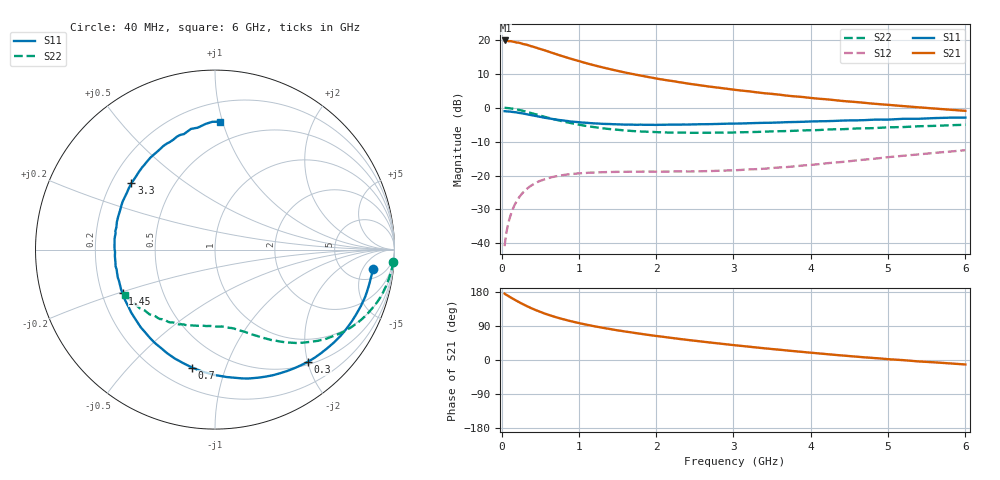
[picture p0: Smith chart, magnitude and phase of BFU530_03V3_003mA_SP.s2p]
! Filename:  P:\Prog\Test\Noise\ATS_data\Testdata_Net\03 Spar\BFU530_APG2013_40_A05_03p3V_003mA_SP_CM01_D.s2p
! Date/Time: Fri 26/Apr/2013 13:03:17
! BFU530_APG2013_40_A05_03p3V_1to25mA_SP_CM01_Bias3_R.s2p
! MDIF S-parameter v. bias file
! BFU530_APG2013_40_A05_03p3V_1to25mA_SP_CM01
! Date/time Wed Apr 24 18:17:07 2013
! VAR V_out= 3.3000
! VAR I_out= 2.9950
! VAR V_in= 0.8102
! VAR I_in= 0.0328
! Device data file deembeded for feedlines and parallel
! Original file: \03 Spar\BFU530_APG2013_40_A05_03p3V_003mA_SP_CM01_R.s2p
! Feed-files: PR047V01_250413_Feed1.s2p, PR047V01_250413_Feed2.s2p
! Parallel-file: PR047V01_250413_Par.s2p
# MHz S MA R 50
!  Freq-MHz  S11-mag  S11-arg  S21-mag  S21-arg  S12-mag  S12-arg  S22-mag  S22-arg
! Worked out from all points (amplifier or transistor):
!   98 points, 40 MHz to 6 GHz, reference 50 ohm
!   highest |S21| = 19.8 dB at 50 MHz (marker M1)
!   |S21| within 3 dB of that: start of sweep to 570 MHz
!   unconditionally stable (mu >= 1): 2.566 GHz to 4.777 GHz
!   at 300 MHz: K = 0.14, MSG = 21.6 dB, |S12| = -24.5 dB
!   at 1.6 GHz: K = 0.67, MSG = 14.6 dB, |S12| = -18.9 dB
!   at 6 GHz: K = 0.85, MSG = 5.8 dB, |S12| = -12.5 dB
!   S11 on the Smith chart (normalised r, x): 40 MHz: 8, -8; 300 MHz: 0.55, -2.00; 700 MHz: 0.32, -0.77; 1.45 GHz: 0.29, -0.21; 3.3 GHz: 0.28, +0.32; 6 GHz: 0.34, +0.98
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40  0.8866 -7.1  9.759 175.1  0.009105 85.7  0.9938 -3.9
50  0.8846 -8.9  9.775 173.1  0.01136 84.5  0.9941 -5.0
70  0.8812 -12.2  9.653 171.3  0.01579 82.9  0.9881 -7.2
120  0.8716 -21.1  9.543 164.9  0.02664 77.8  0.9741 -12.1
220  0.841 -37.9  9.068 153.4  0.04631 68.5  0.9289 -21.5
300  0.8113 -50.5  8.576 145.0  0.0596 61.8  0.8842 -28.2
360  0.7861 -59.5  8.214 139.2  0.0681 57.3  0.8488 -32.8
460  0.7477 -73.2  7.577 130.4  0.07976 50.8  0.7895 -39.3
550  0.7131 -84.7  7.036 123.2  0.08733 45.8  0.7358 -44.4
700  0.6696 -100.9  6.18 113.2  0.09701 39.4  0.6651 -51.2
850  0.636 -114.7  5.453 104.8  0.1035 34.5  0.6071 -56.5
1050  0.6028 -130.4  4.677 95.2  0.1085 29.8  0.5483 -62.7
1200  0.5867 -140.4  4.207 89.0  0.1108 27.2  0.5162 -66.4
1450  0.5693 -154.6  3.593 80.0  0.113 24.3  0.478 -71.7
1750  0.5593 -168.8  3.043 70.6  0.1139 22.6  0.4487 -77.5
2050  0.5595 179.8  2.63 62.2  0.114 22.3  0.4335 -83.1
2450  0.5656 165.5  2.228 51.9  0.1146 23.2  0.4258 -90.5
3100  0.5847 146.8  1.787 37.2  0.1209 27.9  0.4339 -101.8
3300  0.5942 141.6  1.683 33.0  0.1242 29.4  0.439 -105.5
4100  0.6296 122.9  1.355 17.5  0.1469 34.1  0.4678 -119.8
5200  0.6856 101.3  1.053 -0.4  0.1956 34.0  0.5182 -139.2
6000  0.7135 87.9  0.8981 -11.8  0.236 29.5  0.5605 -153.1
